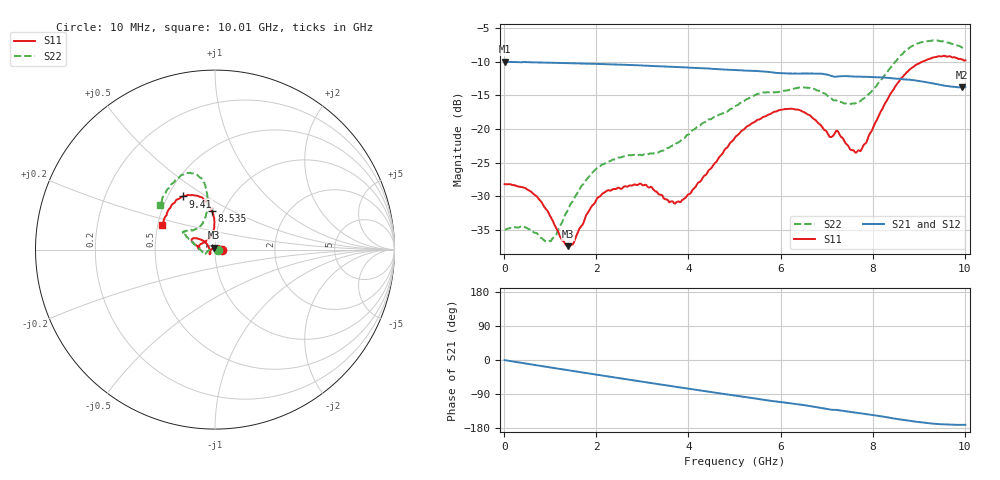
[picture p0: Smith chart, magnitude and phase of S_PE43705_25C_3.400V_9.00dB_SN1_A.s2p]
! Device ID: PE43705
! Serial: 1
! Insertion: A
! Impedance: 50 ohm
! Temp: 25C
! VDD: 3.400V
! Attenuation Step: 9.00dB
#  Hz  S  RI  R  50
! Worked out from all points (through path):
!   401 points, 10 MHz to 10.01 GHz, reference 50 ohm
!   highest |S21| = -10.00 dB at 10 MHz (marker M1); lowest = -13.8 dB at 9.935 GHz (marker M2)
!   group delay of S21, straight-line fit = 49.3 ps
!   lowest |S11| = -37.4 dB at 1.385 GHz (marker M3), VSWR 1.03, Z = 49.3 + j1.14 ohm
!   |S11| at or under -10 dB: start of sweep to 9.073 GHz
!   |S22| runs from -36.7 to -6.8 dB; largest |S21 - S12| = 0.0028
!   S11 on the Smith chart (normalised r, x): 10 MHz: 1.08, +0.00; 8.535 GHz: 0.88, +0.40; 9.41 GHz: 0.60, +0.40; 10.01 GHz: 0.53, +0.16
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1e7  0.0388 0.000173  0.3163 -0.0015  0.3166 -0.00132  0.0178 0.000223
5.35e8  0.0303 0.0176  0.308 -0.0581  0.3081 -0.058  0.0111 0.0141
9.6e8  0.0127 0.0203  0.2946 -0.1007  0.2947 -0.1006  -0.00528 0.0137
1.385e9  -0.0068 0.0116  0.2753 -0.1399  0.2755 -0.1398  -0.0247 0.00387
1.685e9  -0.019 0.00138  0.2584 -0.1654  0.2584 -0.1654  -0.0374 -0.00598
2.21e9  -0.03 -0.0166  0.2233 -0.2051  0.2235 -0.2049  -0.0519 -0.0213
2.96e9  -0.0297 -0.0257  0.163 -0.2481  0.1633 -0.2479  -0.0605 -0.0213
3.36e9  -0.0256 -0.02  0.1283 -0.2633  0.1285 -0.2629  -0.065 -0.0167
3.635e9  -0.0269 -0.0103  0.1037 -0.2711  0.1039 -0.2709  -0.074 -0.00934
3.885e9  -0.0299 0.000784  0.0808 -0.2758  0.0812 -0.2756  -0.0841 0.000601
5.01e9  -0.069 0.0522  -0.0183 -0.2737  -0.0179 -0.2737  -0.1379 0.0528
5.985e9  -0.1239 0.062  -0.0922 -0.2436  -0.0909 -0.2439  -0.1669 0.0892
6.685e9  -0.117 0.0322  -0.139 -0.2177  -0.1391 -0.2174  -0.1708 0.1019
7.06e9  -0.0866 0.0129  -0.163 -0.1902  -0.1626 -0.1911  -0.134 0.1088
7.235e9  -0.0951 0.0182  -0.1647 -0.1825  -0.1639 -0.183  -0.1182 0.1097
7.685e9  -0.0383 0.0578  -0.1873 -0.1587  -0.187 -0.1589  -0.0746 0.1406
8.36e9  -0.00489 0.1765  -0.2119 -0.1119  -0.2107 -0.1127  -0.0412 0.2765
8.535e9  -0.0194 0.2173  -0.2154 -0.0971  -0.2137 -0.0991  -0.0476 0.3259
8.935e9  -0.0719 0.2909  -0.2192 -0.0683  -0.2179 -0.0665  -0.1009 0.4166
9.41e9  -0.1794 0.296  -0.2109 -0.0412  -0.2104 -0.0411  -0.1873 0.4152
9.935e9  -0.2852 0.1649  -0.2011 -0.0315  -0.2023 -0.032  -0.2951 0.2756
1.001e10  -0.294 0.137  -0.2021 -0.0318  -0.2027 -0.033  -0.3078 0.2482
